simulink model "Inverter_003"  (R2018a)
settings: Solver=FixedStepDiscrete  StartTime=0.0  StopTime=inf  RelTol=1e-3  EnableMultiTasking=on
PreLoadFcn:
  | Sample_Time
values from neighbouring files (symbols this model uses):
  C_filt = 4.7e-6 /2  /2    (= 1.175e-06)    [Sample_Time.m]
  L_filt = 10e-3  /2  *2    (= 0.01)    [Sample_Time.m]
  Tcontrol = 5e-5    (= 5e-05)    [Sample_Time.m]
  Tmeasure = 5e-5     *2    (= 0.0001)    [Sample_Time.m]
  Tsample = 1e-6    (= 1e-06)    [Sample_Time.m]
  Tscope = Tcontrol*20    (= 0.001)    [Sample_Time.m]
  w = 2*pi*50    (= 314.159265359)    [Sample_Time.m]
undefined symbols (not defined in the file or in its folder): A, ADCIN0, ADCIN1, ADCINA0, ADCINB0, bit, C_filtEST, Compare, conversion, DCAEVT1, DCAEVT1FILT, Digital, Down, ended, Event, Filtered, GPTRIP1SEL, GPTRIP2SEL, input, Module, of, Single, start, Trip, TZ1, TZ2, Up, version, Zone
libraries: tiiqmathlib x32, simulink x16, c2802xlib x13, c2837xDlib x13, powerlib_meascontrol x4, etargetslib x4, c28xdmclib x1
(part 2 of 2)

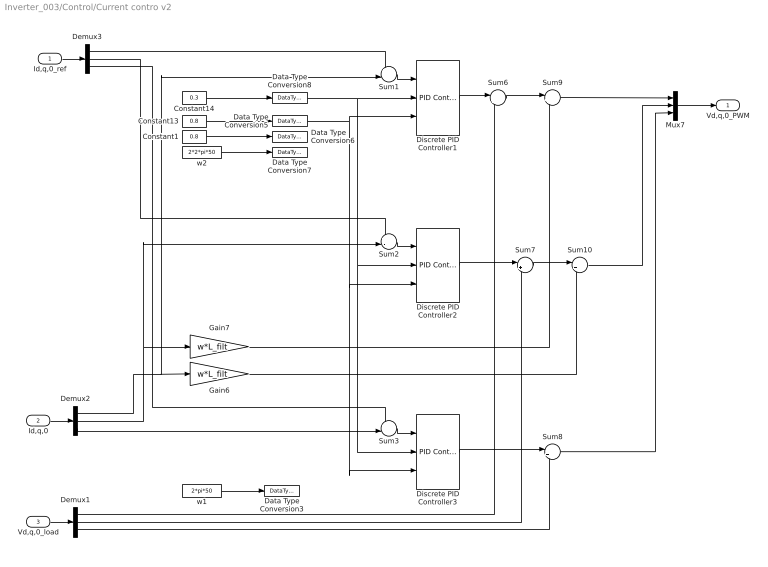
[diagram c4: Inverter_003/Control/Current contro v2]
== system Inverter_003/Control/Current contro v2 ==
  Id,q,0_ref : Inport
  Id,q,0 : Inport  Port=2
  Vd,q,0_load : Inport  Port=3
  Constant1 : Constant  Value=0.8
  Constant13 : Constant  Value=0.8
  Constant14 : Constant  Value=0.3
  Data Type Conversion{3,5..8} (5 alike) : DataTypeConversion  OutDataTypeStr=single
  Demux1 : Demux  Outputs=3
  Demux2 : Demux  Outputs=3
  Demux3 : Demux  Outputs=3
  Discrete PID Controller1 : simulink/Continuous/PID Controller  Controller=PI  TimeDomain=Discrete-time  SampleTime=Tcontrol  IntegratorMethod=Backward Euler  FilterMethod=Forward Euler  Form=Parallel  UseFilter=on  ControllerParametersSource=external  P=1  I=1  D=0  N=100  InitialConditionSource=internal  InitialConditionForIntegrator=0  InitialConditionForFilter=0  ExternalReset=none  LimitOutput=on  UpperSaturationLimit=0.98  LowerSaturationLimit=0  LinearizeAsGain=off  AntiWindupMode=clamping  Kb=1  TrackingMode=off  Kt=1  PParamMin=[]  PParamMax=[]  IParamMin=[]  IParamMax=[]  DParamMin=[]  DParamMax=[]  NParamMin=[]  NParamMax=[]  KbParamMin=[]  KbParamMax=[]  KtParamMin=[]  KtParamMax=[]  POutMin=[]  POutMax=[]  IOutMin=[]  IOutMax=[]  DOutMin=[]  DOutMax=[]  NOutMin=[]  NOutMax=[]  KbOutMin=[]  KbOutMax=[]  KtOutMin=[]  KtOutMax=[]  IntegratorOutMin=[]  IntegratorOutMax=[]  FilterOutMin=[]  FilterOutMax=[]  SumOutMin=[]  SumOutMax=[]  SumI1OutMin=[]  SumI1OutMax=[]  SumI2OutMin=[]  SumI2OutMax=[]  SumI3OutMin=[]  SumI3OutMax=[]  SumDOutMin=[]  SumDOutMax=[]  SaturationOutMin=[]  SaturationOutMax=[]  IntegratorContinuousStateAttributes=''  IntegratorStateMustResolveToSignalObject=off  IntegratorRTWStateStorageClass=Auto  FilterContinuousStateAttributes=''  FilterStateMustResolveToSignalObject=off  FilterRTWStateStorageClass=Auto  DifferentiatorICPrevScaledInput=0  DifferentiatorOutMin=[]  DifferentiatorOutMax=[]  FilterDiffOutCoefMin=[]  FilterDiffOutCoefMax=[]  SumDenOutMin=[]  SumDenOutMax=[]  SumNumOutMin=[]  SumNumOutMax=[]  ReciprocalOutMin=[]  ReciprocalOutMax=[]  DivideOutMin=[]  DivideOutMax=[]  TunerSelectOption=Transfer Function Based (PID Tuner App)
  Discrete PID Controller2 : simulink/Continuous/PID Controller  Controller=PI  TimeDomain=Discrete-time  SampleTime=Tcontrol  IntegratorMethod=Backward Euler  FilterMethod=Forward Euler  Form=Parallel  UseFilter=on  ControllerParametersSource=external  P=1  I=1  D=0  N=100  InitialConditionSource=internal  InitialConditionForIntegrator=0  InitialConditionForFilter=0  ExternalReset=none  LimitOutput=on  UpperSaturationLimit=0.98  LowerSaturationLimit=0  LinearizeAsGain=off  AntiWindupMode=clamping  Kb=1  TrackingMode=off  Kt=1  PParamMin=[]  PParamMax=[]  IParamMin=[]  IParamMax=[]  DParamMin=[]  DParamMax=[]  NParamMin=[]  NParamMax=[]  KbParamMin=[]  KbParamMax=[]  KtParamMin=[]  KtParamMax=[]  POutMin=[]  POutMax=[]  IOutMin=[]  IOutMax=[]  DOutMin=[]  DOutMax=[]  NOutMin=[]  NOutMax=[]  KbOutMin=[]  KbOutMax=[]  KtOutMin=[]  KtOutMax=[]  IntegratorOutMin=[]  IntegratorOutMax=[]  FilterOutMin=[]  FilterOutMax=[]  SumOutMin=[]  SumOutMax=[]  SumI1OutMin=[]  SumI1OutMax=[]  SumI2OutMin=[]  SumI2OutMax=[]  SumI3OutMin=[]  SumI3OutMax=[]  SumDOutMin=[]  SumDOutMax=[]  SaturationOutMin=[]  SaturationOutMax=[]  IntegratorContinuousStateAttributes=''  IntegratorStateMustResolveToSignalObject=off  IntegratorRTWStateStorageClass=Auto  FilterContinuousStateAttributes=''  FilterStateMustResolveToSignalObject=off  FilterRTWStateStorageClass=Auto  DifferentiatorICPrevScaledInput=0  DifferentiatorOutMin=[]  DifferentiatorOutMax=[]  FilterDiffOutCoefMin=[]  FilterDiffOutCoefMax=[]  SumDenOutMin=[]  SumDenOutMax=[]  SumNumOutMin=[]  SumNumOutMax=[]  ReciprocalOutMin=[]  ReciprocalOutMax=[]  DivideOutMin=[]  DivideOutMax=[]  TunerSelectOption=Transfer Function Based (PID Tuner App)
  Discrete PID Controller3 : simulink/Continuous/PID Controller  Controller=PI  TimeDomain=Discrete-time  SampleTime=Tcontrol  IntegratorMethod=Backward Euler  FilterMethod=Forward Euler  Form=Parallel  UseFilter=on  ControllerParametersSource=external  P=1  I=1  D=0  N=100  InitialConditionSource=internal  InitialConditionForIntegrator=0  InitialConditionForFilter=0  ExternalReset=none  LimitOutput=on  UpperSaturationLimit=0.98  LowerSaturationLimit=0  LinearizeAsGain=off  AntiWindupMode=clamping  Kb=1  TrackingMode=off  Kt=1  PParamMin=[]  PParamMax=[]  IParamMin=[]  IParamMax=[]  DParamMin=[]  DParamMax=[]  NParamMin=[]  NParamMax=[]  KbParamMin=[]  KbParamMax=[]  KtParamMin=[]  KtParamMax=[]  POutMin=[]  POutMax=[]  IOutMin=[]  IOutMax=[]  DOutMin=[]  DOutMax=[]  NOutMin=[]  NOutMax=[]  KbOutMin=[]  KbOutMax=[]  KtOutMin=[]  KtOutMax=[]  IntegratorOutMin=[]  IntegratorOutMax=[]  FilterOutMin=[]  FilterOutMax=[]  SumOutMin=[]  SumOutMax=[]  SumI1OutMin=[]  SumI1OutMax=[]  SumI2OutMin=[]  SumI2OutMax=[]  SumI3OutMin=[]  SumI3OutMax=[]  SumDOutMin=[]  SumDOutMax=[]  SaturationOutMin=[]  SaturationOutMax=[]  IntegratorContinuousStateAttributes=''  IntegratorStateMustResolveToSignalObject=off  IntegratorRTWStateStorageClass=Auto  FilterContinuousStateAttributes=''  FilterStateMustResolveToSignalObject=off  FilterRTWStateStorageClass=Auto  DifferentiatorICPrevScaledInput=0  DifferentiatorOutMin=[]  DifferentiatorOutMax=[]  FilterDiffOutCoefMin=[]  FilterDiffOutCoefMax=[]  SumDenOutMin=[]  SumDenOutMax=[]  SumNumOutMin=[]  SumNumOutMax=[]  ReciprocalOutMin=[]  ReciprocalOutMax=[]  DivideOutMin=[]  DivideOutMax=[]  TunerSelectOption=Transfer Function Based (PID Tuner App)
  Gain6 : Gain  Gain=w*L_filt
  Gain7 : Gain  Gain=w*L_filt
  Mux7 : Mux  Inputs=3
  Sum1 : Sum  Inputs=+-|
  Sum{6..8,10} (4 alike) : Sum  Inputs=|++
  Sum2 : Sum  Inputs=+-|
  Sum3 : Sum  Inputs=+-|
  Sum9 : Sum  Inputs=|+-
  w1 : Constant  Value=2*pi*50  OutDataTypeStr=fixdt(1,32,2^-15,0)  SampleTime=-1
  w2 : Constant  Value=2*2*pi*50  OutMin=[1e-4]  OutMax=[1000]  OutDataTypeStr=fixdt(1,32,2^-15,0)  SampleTime=-1
  Vd,q,0_PWM : Outport
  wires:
  Sum8/1 -> Mux7/3
  Discrete PID Controller2/1 -> Sum7/1
  Demux1/3 -> Sum8/2
  Demux3/3 -> Sum3/1
  Discrete PID Controller3/1 -> Sum8/1
  Demux1/1 -> Sum6/2
  Demux1/2 -> Sum7/2
  Sum6/1 -> Sum9/1
  Sum9/1 -> Mux7/1
  Sum7/1 -> Sum10/1
  Sum10/1 -> Mux7/2
  Gain7/1 -> Sum9/2
  Demux3/1 -> Sum1/1
  Demux3/2 -> Sum2/1
  Id,q,0/1 -> Demux2/1
  Id,q,0_ref/1 -> Demux3/1
  Vd,q,0_load/1 -> Demux1/1
  Demux2/2 -> Sum2/2, Gain7/1
  Demux2/1 -> Sum1/2, Gain6/1
  Mux7/1 -> Vd,q,0_PWM/1
  w1/1 -> Data Type Conversion3/1
  Constant14/1 -> Data Type Conversion8/1
  w2/1 -> Data Type Conversion7/1
  Constant13/1 -> Data Type Conversion5/1
  Constant1/1 -> Data Type Conversion6/1
  Gain6/1 -> Sum10/2
  Discrete PID Controller1/1 -> Sum6/1
  Data Type Conversion5/1 -> Discrete PID Controller1/3, Discrete PID Controller2/3, Discrete PID Controller3/3
  Data Type Conversion8/1 -> Discrete PID Controller1/2, Discrete PID Controller2/2, Discrete PID Controller3/2
  Sum1/1 -> Discrete PID Controller1/1
  Sum2/1 -> Discrete PID Controller2/1
  Sum3/1 -> Discrete PID Controller3/1
  Demux2/3 -> Sum3/2

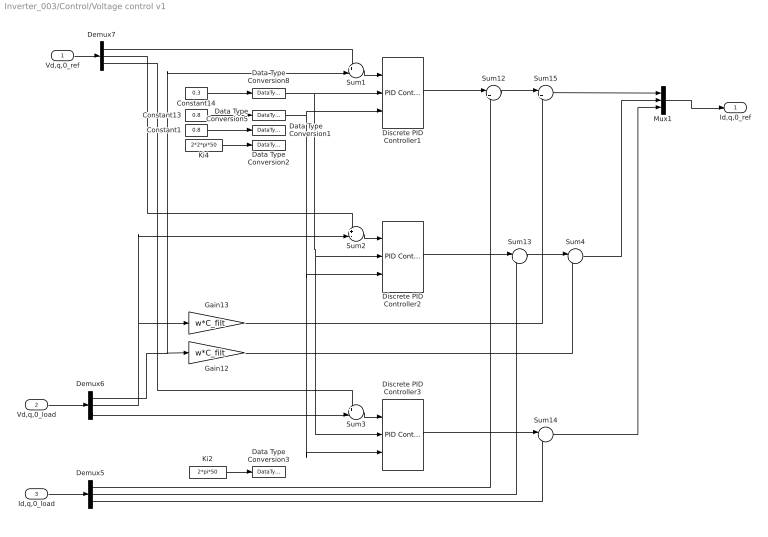
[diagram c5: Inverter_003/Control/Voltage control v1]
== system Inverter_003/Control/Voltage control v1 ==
  Vd,q,0_ref : Inport
  Vd,q,0_load : Inport  Port=2
  Id,q,0_load : Inport  Port=3
  Constant1 : Constant  Value=0.8
  Constant13 : Constant  Value=0.8
  Constant14 : Constant  Value=0.3
  Data Type Conversion{1..3,5,8} (5 alike) : DataTypeConversion  OutDataTypeStr=single
  Demux5 : Demux  Outputs=3
  Demux6 : Demux  Outputs=3
  Demux7 : Demux  Outputs=3
  Discrete PID Controller1 : simulink/Continuous/PID Controller  Controller=PI  TimeDomain=Discrete-time  SampleTime=Tcontrol  IntegratorMethod=Backward Euler  FilterMethod=Forward Euler  Form=Parallel  UseFilter=on  ControllerParametersSource=external  P=1  I=1  D=0  N=100  InitialConditionSource=internal  InitialConditionForIntegrator=0  InitialConditionForFilter=0  ExternalReset=none  LimitOutput=on  UpperSaturationLimit=0.98  LowerSaturationLimit=0  LinearizeAsGain=off  AntiWindupMode=clamping  Kb=1  TrackingMode=off  Kt=1  PParamMin=[]  PParamMax=[]  IParamMin=[]  IParamMax=[]  DParamMin=[]  DParamMax=[]  NParamMin=[]  NParamMax=[]  KbParamMin=[]  KbParamMax=[]  KtParamMin=[]  KtParamMax=[]  POutMin=[]  POutMax=[]  IOutMin=[]  IOutMax=[]  DOutMin=[]  DOutMax=[]  NOutMin=[]  NOutMax=[]  KbOutMin=[]  KbOutMax=[]  KtOutMin=[]  KtOutMax=[]  IntegratorOutMin=[]  IntegratorOutMax=[]  FilterOutMin=[]  FilterOutMax=[]  SumOutMin=[]  SumOutMax=[]  SumI1OutMin=[]  SumI1OutMax=[]  SumI2OutMin=[]  SumI2OutMax=[]  SumI3OutMin=[]  SumI3OutMax=[]  SumDOutMin=[]  SumDOutMax=[]  SaturationOutMin=[]  SaturationOutMax=[]  IntegratorContinuousStateAttributes=''  IntegratorStateMustResolveToSignalObject=off  IntegratorRTWStateStorageClass=Auto  FilterContinuousStateAttributes=''  FilterStateMustResolveToSignalObject=off  FilterRTWStateStorageClass=Auto  DifferentiatorICPrevScaledInput=0  DifferentiatorOutMin=[]  DifferentiatorOutMax=[]  FilterDiffOutCoefMin=[]  FilterDiffOutCoefMax=[]  SumDenOutMin=[]  SumDenOutMax=[]  SumNumOutMin=[]  SumNumOutMax=[]  ReciprocalOutMin=[]  ReciprocalOutMax=[]  DivideOutMin=[]  DivideOutMax=[]  TunerSelectOption=Transfer Function Based (PID Tuner App)
  Discrete PID Controller2 : simulink/Continuous/PID Controller  Controller=PI  TimeDomain=Discrete-time  SampleTime=Tcontrol  IntegratorMethod=Backward Euler  FilterMethod=Forward Euler  Form=Parallel  UseFilter=on  ControllerParametersSource=external  P=1  I=1  D=0  N=100  InitialConditionSource=internal  InitialConditionForIntegrator=0  InitialConditionForFilter=0  ExternalReset=none  LimitOutput=on  UpperSaturationLimit=0.98  LowerSaturationLimit=0  LinearizeAsGain=off  AntiWindupMode=clamping  Kb=1  TrackingMode=off  Kt=1  PParamMin=[]  PParamMax=[]  IParamMin=[]  IParamMax=[]  DParamMin=[]  DParamMax=[]  NParamMin=[]  NParamMax=[]  KbParamMin=[]  KbParamMax=[]  KtParamMin=[]  KtParamMax=[]  POutMin=[]  POutMax=[]  IOutMin=[]  IOutMax=[]  DOutMin=[]  DOutMax=[]  NOutMin=[]  NOutMax=[]  KbOutMin=[]  KbOutMax=[]  KtOutMin=[]  KtOutMax=[]  IntegratorOutMin=[]  IntegratorOutMax=[]  FilterOutMin=[]  FilterOutMax=[]  SumOutMin=[]  SumOutMax=[]  SumI1OutMin=[]  SumI1OutMax=[]  SumI2OutMin=[]  SumI2OutMax=[]  SumI3OutMin=[]  SumI3OutMax=[]  SumDOutMin=[]  SumDOutMax=[]  SaturationOutMin=[]  SaturationOutMax=[]  IntegratorContinuousStateAttributes=''  IntegratorStateMustResolveToSignalObject=off  IntegratorRTWStateStorageClass=Auto  FilterContinuousStateAttributes=''  FilterStateMustResolveToSignalObject=off  FilterRTWStateStorageClass=Auto  DifferentiatorICPrevScaledInput=0  DifferentiatorOutMin=[]  DifferentiatorOutMax=[]  FilterDiffOutCoefMin=[]  FilterDiffOutCoefMax=[]  SumDenOutMin=[]  SumDenOutMax=[]  SumNumOutMin=[]  SumNumOutMax=[]  ReciprocalOutMin=[]  ReciprocalOutMax=[]  DivideOutMin=[]  DivideOutMax=[]  TunerSelectOption=Transfer Function Based (PID Tuner App)
  Discrete PID Controller3 : simulink/Continuous/PID Controller  Controller=PI  TimeDomain=Discrete-time  SampleTime=Tcontrol  IntegratorMethod=Backward Euler  FilterMethod=Forward Euler  Form=Parallel  UseFilter=on  ControllerParametersSource=external  P=1  I=1  D=0  N=100  InitialConditionSource=internal  InitialConditionForIntegrator=0  InitialConditionForFilter=0  ExternalReset=none  LimitOutput=on  UpperSaturationLimit=0.98  LowerSaturationLimit=0  LinearizeAsGain=off  AntiWindupMode=clamping  Kb=1  TrackingMode=off  Kt=1  PParamMin=[]  PParamMax=[]  IParamMin=[]  IParamMax=[]  DParamMin=[]  DParamMax=[]  NParamMin=[]  NParamMax=[]  KbParamMin=[]  KbParamMax=[]  KtParamMin=[]  KtParamMax=[]  POutMin=[]  POutMax=[]  IOutMin=[]  IOutMax=[]  DOutMin=[]  DOutMax=[]  NOutMin=[]  NOutMax=[]  KbOutMin=[]  KbOutMax=[]  KtOutMin=[]  KtOutMax=[]  IntegratorOutMin=[]  IntegratorOutMax=[]  FilterOutMin=[]  FilterOutMax=[]  SumOutMin=[]  SumOutMax=[]  SumI1OutMin=[]  SumI1OutMax=[]  SumI2OutMin=[]  SumI2OutMax=[]  SumI3OutMin=[]  SumI3OutMax=[]  SumDOutMin=[]  SumDOutMax=[]  SaturationOutMin=[]  SaturationOutMax=[]  IntegratorContinuousStateAttributes=''  IntegratorStateMustResolveToSignalObject=off  IntegratorRTWStateStorageClass=Auto  FilterContinuousStateAttributes=''  FilterStateMustResolveToSignalObject=off  FilterRTWStateStorageClass=Auto  DifferentiatorICPrevScaledInput=0  DifferentiatorOutMin=[]  DifferentiatorOutMax=[]  FilterDiffOutCoefMin=[]  FilterDiffOutCoefMax=[]  SumDenOutMin=[]  SumDenOutMax=[]  SumNumOutMin=[]  SumNumOutMax=[]  ReciprocalOutMin=[]  ReciprocalOutMax=[]  DivideOutMin=[]  DivideOutMax=[]  TunerSelectOption=Transfer Function Based (PID Tuner App)
  Gain12 : Gain  Gain=w*C_filt
  Gain13 : Gain  Gain=w*C_filt
  Ki2 : Constant  Value=2*pi*50  OutDataTypeStr=fixdt(1,32,2^-10,0)  SampleTime=-1
  Ki4 : Constant  Value=2*2*pi*50  OutDataTypeStr=fixdt(1,32,2^-10,0)  SampleTime=-1
  Mux1 : Mux  Inputs=3
  Sum1 : Sum  Inputs=+-|
  Sum{4,12..14} (4 alike) : Sum  Inputs=|++
  Sum15 : Sum  Inputs=|+-
  Sum2 : Sum  Inputs=+-|
  Sum3 : Sum  Inputs=+-|
  Id,q,0_ref : Outport
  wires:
  Vd,q,0_load/1 -> Demux6/1
  Vd,q,0_ref/1 -> Demux7/1
  Id,q,0_load/1 -> Demux5/1
  Demux6/1 -> Sum1/2, Gain12/1
  Demux6/2 -> Sum2/2, Gain13/1
  Demux7/2 -> Sum2/1
  Demux7/1 -> Sum1/1
  Gain13/1 -> Sum15/2
  Gain12/1 -> Sum4/2
  Sum4/1 -> Mux1/2
  Sum13/1 -> Sum4/1
  Sum15/1 -> Mux1/1
  Sum12/1 -> Sum15/1
  Demux5/2 -> Sum13/2
  Demux5/1 -> Sum12/2
  Discrete PID Controller1/1 -> Sum12/1
  Discrete PID Controller3/1 -> Sum14/1
  Demux6/3 -> Sum3/2
  Demux7/3 -> Sum3/1
  Demux5/3 -> Sum14/2
  Discrete PID Controller2/1 -> Sum13/1
  Sum14/1 -> Mux1/3
  Mux1/1 -> Id,q,0_ref/1
  Constant13/1 -> Data Type Conversion5/1
  Data Type Conversion8/1 -> Discrete PID Controller1/2, Discrete PID Controller3/2, Discrete PID Controller2/2
  Data Type Conversion5/1 -> Discrete PID Controller1/3, Discrete PID Controller3/3, Discrete PID Controller2/3
  Constant1/1 -> Data Type Conversion1/1
  Ki4/1 -> Data Type Conversion2/1
  Ki2/1 -> Data Type Conversion3/1
  Sum1/1 -> Discrete PID Controller1/1
  Sum2/1 -> Discrete PID Controller2/1
  Sum3/1 -> Discrete PID Controller3/1
  Constant14/1 -> Data Type Conversion8/1

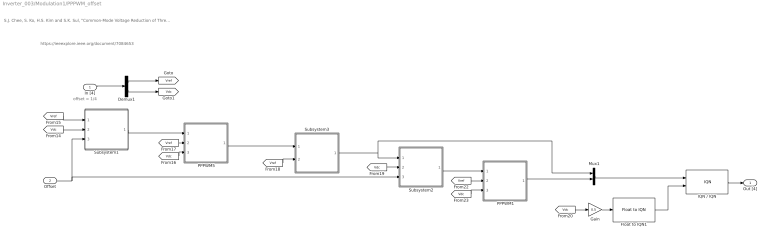
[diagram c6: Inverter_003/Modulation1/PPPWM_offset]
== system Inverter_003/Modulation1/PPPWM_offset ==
  note: offset = 1/4
  note: https://ieeexplore.ieee.org/document/7084653
  note: S.J. Chee, S. Ko, H.S. Kim and S.K. Sul, "Common-Mode Voltage Reduction of Three-Level Four-Leg PWM Converter", IEEE Transactions on Industry Applications, vol. 51, no. 5, Sept.-Oct. 2015, pp. 4006-4016
  In [4] : Inport
  Offset : Inport  Port=2
  Demux1 : Demux  Outputs=[3 1]
  Float to IQN1 : tiiqmathlib/Float to IQN  Q_value=10
  Gain : Gain  Gain=0.5  OutDataTypeStr=single
  IQN / IQN : tiiqmathlib/IQN // IQN
  Mux1 : Mux  Inputs=2
  PPPWM1 : Subsystem  TreatAsAtomicUnit=on
  PPPWM5 : Subsystem  TreatAsAtomicUnit=on
  Subsystem1 : Subsystem  TreatAsAtomicUnit=on
  Subsystem2 : Subsystem  TreatAsAtomicUnit=on
  Subsystem3 : Subsystem  TreatAsAtomicUnit=on
  Out [4] : Outport
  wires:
  Subsystem3/1(Vref *) -> Subsystem2/1(Voltage), Mux1/1
  PPPWM1/1(Vfn) -> Mux1/2
  Mux1/1 -> IQN / IQN/1
  IQN / IQN/1 -> Out [4]/1
  [Vdc] -> Gain/1
  [Vdc] -> PPPWM1/3(Vdc)
  [Vref] -> PPPWM1/2(Vref)
  Subsystem2/1(Voltage+Offset) -> PPPWM1/1(Voffset)
  PPPWM5/1(Vfn) -> Subsystem3/1(Vfn)
  [Vdc] -> Subsystem2/2(Vdc)
  [Vref] -> Subsystem3/2(Vref)
  [Vdc] -> PPPWM5/3(Vdc)
  [Vref] -> PPPWM5/2(Vref)
  [Vdc] -> Subsystem1/2(Vdc)
  [Vref] -> Subsystem1/1(Voltage)
  Demux1/2 -> [Vdc]
  Demux1/1 -> [Vref]
  Offset/1 -> Subsystem2/3(Offset), Subsystem1/3(Offset)
  In [4]/1 -> Demux1/1
  Gain/1 -> Float to IQN1/1
  Float to IQN1/1 -> IQN / IQN/2
  Subsystem1/1(Voltage+Offset) -> PPPWM5/1(Voffset)

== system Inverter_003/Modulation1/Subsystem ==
  note: Carrier
  Vref : Inport
  Add1 : Sum  Inputs=|++
  Constant : Constant  Value=-0.5  OutDataTypeStr=fixdt(1,32,2^-10,0)
  IQN1 x IQN2 : tiiqmathlib/IQN1 x IQN2  Q=10
  MinMax : MinMax  ZeroCross=off
  MinMax1 : MinMax  Function=max  ZeroCross=off
  Mux1 : Mux  Inputs=2
  Sum : Sum  Inputs=|++
  Out[4] : Outport
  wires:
  IQN1 x IQN2/1 -> Add1/2, Mux1/2  "PhaseN"
  Add1/1 -> Mux1/1
  Mux1/1 -> Out[4]/1
  Constant/1 -> IQN1 x IQN2/2
  Sum/1 -> IQN1 x IQN2/1
  Vref/1 -> MinMax/1, MinMax1/1, Add1/1
  MinMax1/1 -> Sum/2
  MinMax/1 -> Sum/1

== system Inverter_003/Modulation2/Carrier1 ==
  In1 : Inport
  Gain : Gain  Gain=-0.5
  Gain1 : Gain  Gain=-0.5
  MATLAB Function : MATLAB Function  Commented=on  TreatAsAtomicUnit=on
  MinMax : MinMax  ZeroCross=off
  MinMax1 : MinMax  Function=max  ZeroCross=off
  Sum : Sum  Inputs=|++
  Out1 : Outport
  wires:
  Sum/1 -> Out1/1
  In1/1 -> MinMax1/1, MinMax/1
  Gain1/1 -> Sum/2
  Gain/1 -> Sum/1
  MinMax1/1 -> Gain1/1, MATLAB Function/2(In2)
  MinMax/1 -> Gain/1, MATLAB Function/1(In1)

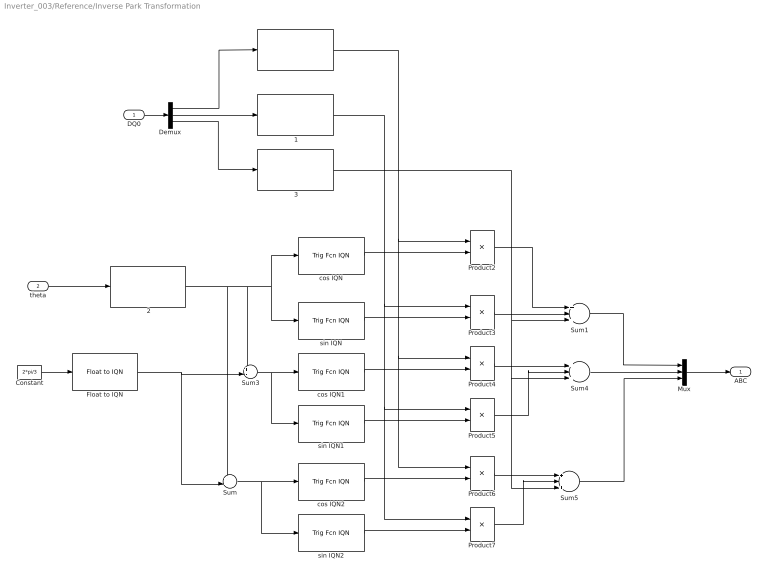
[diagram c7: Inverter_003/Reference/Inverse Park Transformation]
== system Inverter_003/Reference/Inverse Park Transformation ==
  DQ0 : Inport
  theta : Inport  Port=2
   {,1..3} (4 alike) : etargetslib/ 
  Constant : Constant  Value=2*pi/3  OutDataTypeStr=single  SampleTime=0.1
  Demux : Demux  Outputs=3
  Float to IQN : tiiqmathlib/Float to IQN  Q_value=10
  Mux : Mux  Inputs=3
  Product{2..7} (6 alike) : Product
  Sum : Sum  Inputs=++|
  Sum1 : Sum  Inputs=+-+
  Sum3 : Sum  Inputs=+-|
  Sum4 : Sum  Inputs=+-+
  Sum5 : Sum  Inputs=+-+
  cos IQN : tiiqmathlib/Trig Fcn IQN  functionOption=_IQcos
  cos IQN1 : tiiqmathlib/Trig Fcn IQN  functionOption=_IQcos
  cos IQN2 : tiiqmathlib/Trig Fcn IQN  functionOption=_IQcos
  sin IQN : tiiqmathlib/Trig Fcn IQN  functionOption=_IQsin
  sin IQN1 : tiiqmathlib/Trig Fcn IQN  functionOption=_IQsin
  sin IQN2 : tiiqmathlib/Trig Fcn IQN  functionOption=_IQsin
  ABC : Outport
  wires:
  " 2"/1 -> sin IQN/1, cos IQN/1, Sum3/1, Sum/1
  " 1"/1 -> Product7/1, Product5/1, Product3/1
  Product2/1 -> Sum1/1
  Product3/1 -> Sum1/2
  sin IQN/1 -> Product3/2
  cos IQN/1 -> Product2/2
  Demux/2 -> " 1"/1
  Demux/1 -> " "/1
  theta/1 -> " 2"/1
  Demux/3 -> " 3"/1
  Constant/1 -> Float to IQN/1
  Float to IQN/1 -> Sum/2, Sum3/2
  " 3"/1 -> Sum5/3, Sum4/3, Sum1/3
  Sum3/1 -> sin IQN1/1, cos IQN1/1
  cos IQN1/1 -> Product4/2
  sin IQN1/1 -> Product5/2
  Product4/1 -> Sum4/1
  Product5/1 -> Sum4/2
  Sum4/1 -> Mux/2
  Sum/1 -> sin IQN2/1, cos IQN2/1
  " "/1 -> Product2/1, Product4/1, Product6/1
  cos IQN2/1 -> Product6/2
  sin IQN2/1 -> Product7/2
  Product6/1 -> Sum5/1
  Product7/1 -> Sum5/2
  Sum5/1 -> Mux/3
  DQ0/1 -> Demux/1
  Sum1/1 -> Mux/1
  Mux/1 -> ABC/1

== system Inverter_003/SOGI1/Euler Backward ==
  In : Inport
  Gain1 : Gain
  Gain4 : Gain  Gain=SampleTime
  Saturation : Saturate  UpperLimit=UpperLimit  LowerLimit=LowerLimit
  Sum2 : Sum  Inputs=-+
  Sum3 : Sum  Inputs=|++
  Sum5 : Sum  Inputs=|++
  Unit Delay1 : UnitDelay  SampleTime=-1
  Unit Delay2 : UnitDelay  SampleTime=-1
  Out : Outport
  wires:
  Sum5/1 -> Saturation/1, Sum2/1, Unit Delay2/1
  Sum2/1 -> Unit Delay1/1
  Gain4/1 -> Sum3/1
  Unit Delay1/1 -> Gain1/1
  In/1 -> Gain4/1
  Saturation/1 -> Out/1, Sum2/2
  Gain1/1 -> Sum3/2
  Sum3/1 -> Sum5/1
  Unit Delay2/1 -> Sum5/2

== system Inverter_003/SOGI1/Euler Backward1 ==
  In : Inport
  Gain1 : Gain
  Gain4 : Gain  Gain=SampleTime
  Saturation : Saturate  UpperLimit=UpperLimit  LowerLimit=LowerLimit
  Sum2 : Sum  Inputs=-+
  Sum3 : Sum  Inputs=|++
  Sum5 : Sum  Inputs=|++
  Unit Delay1 : UnitDelay  SampleTime=-1
  Unit Delay2 : UnitDelay  SampleTime=-1
  Out : Outport
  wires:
  Unit Delay2/1 -> Sum5/2
  Sum3/1 -> Sum5/1
  Gain1/1 -> Sum3/2
  Saturation/1 -> Sum2/2, Out/1
  In/1 -> Gain4/1
  Unit Delay1/1 -> Gain1/1
  Gain4/1 -> Sum3/1
  Sum2/1 -> Unit Delay1/1
  Sum5/1 -> Unit Delay2/1, Sum2/1, Saturation/1

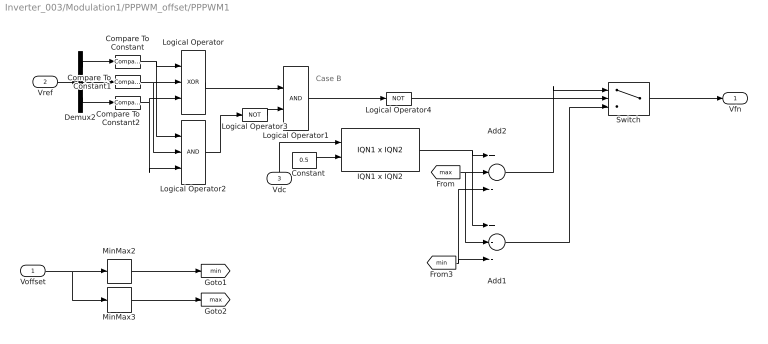
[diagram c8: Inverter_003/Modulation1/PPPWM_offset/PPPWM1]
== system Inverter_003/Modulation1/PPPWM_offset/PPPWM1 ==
  note: Case B
  Voffset : Inport
  Vref : Inport  Port=2
  Vdc : Inport  Port=3
  Add1 : Sum  Inputs=+--
  Add2 : Sum  Inputs=+--
  Compare To Constant : simulink/Logic and Bit Operations/Compare To Constant  relop=>=  const=0  OutDataTypeStr=boolean
  Compare To Constant1 : simulink/Logic and Bit Operations/Compare To Constant  relop=>=  const=0  OutDataTypeStr=boolean
  Compare To Constant2 : simulink/Logic and Bit Operations/Compare To Constant  relop=>=  const=0  OutDataTypeStr=boolean
  Constant : Constant  Value=0.5  OutDataTypeStr=fixdt(1,32,2^-10,0)
  Demux2 : Demux  Outputs=3
  IQN1 x IQN2 : tiiqmathlib/IQN1 x IQN2  Q=10
  Logical Operator : Logic  Operator=XOR  Inputs=3  AllPortsSameDT=off  OutDataTypeStr=boolean
  Logical Operator1 : Logic  AllPortsSameDT=off  OutDataTypeStr=boolean
  Logical Operator2 : Logic  Inputs=3  AllPortsSameDT=off  OutDataTypeStr=boolean
  Logical Operator3 : Logic  Operator=NOT  AllPortsSameDT=off  OutDataTypeStr=boolean
  Logical Operator4 : Logic  Operator=NOT  AllPortsSameDT=off  OutDataTypeStr=boolean
  MinMax2 : MinMax
  MinMax3 : MinMax  Function=max
  Switch : Switch  Criteria=u2 > Threshold
  Vfn : Outport
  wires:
  Switch/1 -> Vfn/1
  Constant/1 -> IQN1 x IQN2/2
  Demux2/3 -> Compare To Constant2/1
  Demux2/2 -> Compare To Constant1/1
  Demux2/1 -> Compare To Constant/1
  Compare To Constant1/1 -> Logical Operator2/2, Logical Operator/2
  MinMax3/1 -> [max]
  MinMax2/1 -> [min]
  Voffset/1 -> MinMax3/1, MinMax2/1
  Vref/1 -> Demux2/1
  Vdc/1 -> IQN1 x IQN2/1
  Compare To Constant/1 -> Logical Operator2/1, Logical Operator/1
  Logical Operator2/1 -> Logical Operator3/1
  Logical Operator1/1 -> Logical Operator4/1
  Compare To Constant2/1 -> Logical Operator2/3, Logical Operator/3
  Add1/1 -> Switch/3
  [max] -> Add1/2, Add2/2
  Add2/1 -> Switch/1
  Logical Operator3/1 -> Logical Operator1/2
  [min] -> Add2/3, Add1/3
  Logical Operator/1 -> Logical Operator1/1
  Logical Operator4/1 -> Switch/2
  IQN1 x IQN2/1 -> Add2/1, Add1/1

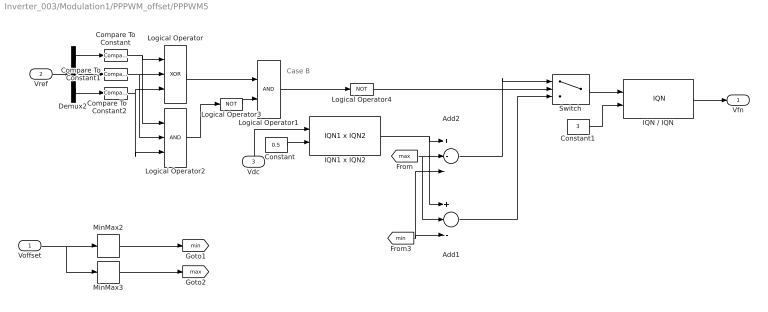
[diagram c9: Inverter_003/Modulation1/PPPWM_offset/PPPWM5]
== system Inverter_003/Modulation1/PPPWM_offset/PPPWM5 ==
  note: Case B
  Voffset : Inport
  Vref : Inport  Port=2
  Vdc : Inport  Port=3
  Add1 : Sum  Inputs=+--
  Add2 : Sum  Inputs=+--
  Compare To Constant : simulink/Logic and Bit Operations/Compare To Constant  relop=>=  const=0  OutDataTypeStr=boolean
  Compare To Constant1 : simulink/Logic and Bit Operations/Compare To Constant  relop=>=  const=0  OutDataTypeStr=boolean
  Compare To Constant2 : simulink/Logic and Bit Operations/Compare To Constant  relop=>=  const=0  OutDataTypeStr=boolean
  Constant : Constant  Value=0.5  OutDataTypeStr=fixdt(1,32,2^-10,0)
  Constant1 : Constant  Value=3  OutDataTypeStr=fixdt(1,32,2^-10,0)
  Demux2 : Demux  Outputs=3
  IQN / IQN : tiiqmathlib/IQN // IQN
  IQN1 x IQN2 : tiiqmathlib/IQN1 x IQN2  Q=10
  Logical Operator : Logic  Operator=XOR  Inputs=3  AllPortsSameDT=off  OutDataTypeStr=boolean
  Logical Operator1 : Logic  AllPortsSameDT=off  OutDataTypeStr=boolean
  Logical Operator2 : Logic  Inputs=3  AllPortsSameDT=off  OutDataTypeStr=boolean
  Logical Operator3 : Logic  Operator=NOT  AllPortsSameDT=off  OutDataTypeStr=boolean
  Logical Operator4 : Logic  Operator=NOT  AllPortsSameDT=off  OutDataTypeStr=boolean
  MinMax2 : MinMax
  MinMax3 : MinMax  Function=max
  Switch : Switch  Criteria=u2 > Threshold
  Vfn : Outport
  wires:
  IQN1 x IQN2/1 -> Add1/1, Add2/1
  Logical Operator4/1 -> Switch/2
  Logical Operator/1 -> Logical Operator1/1
  [min] -> Add1/3, Add2/3
  Logical Operator3/1 -> Logical Operator1/2
  Add2/1 -> Switch/1
  [max] -> Add2/2, Add1/2
  Add1/1 -> Switch/3
  Compare To Constant2/1 -> Logical Operator/3, Logical Operator2/3
  Logical Operator1/1 -> Logical Operator4/1
  Logical Operator2/1 -> Logical Operator3/1
  Compare To Constant/1 -> Logical Operator/1, Logical Operator2/1
  Vdc/1 -> IQN1 x IQN2/1
  Vref/1 -> Demux2/1
  Voffset/1 -> MinMax2/1, MinMax3/1
  Switch/1 -> IQN / IQN/1
  MinMax2/1 -> [min]
  MinMax3/1 -> [max]
  Compare To Constant1/1 -> Logical Operator/2, Logical Operator2/2
  Demux2/1 -> Compare To Constant/1
  Demux2/2 -> Compare To Constant1/1
  Demux2/3 -> Compare To Constant2/1
  Constant/1 -> IQN1 x IQN2/2
  IQN / IQN/1 -> Vfn/1
  Constant1/1 -> IQN / IQN/2

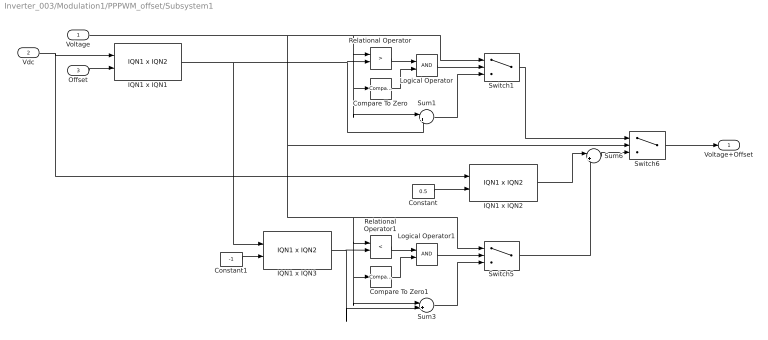
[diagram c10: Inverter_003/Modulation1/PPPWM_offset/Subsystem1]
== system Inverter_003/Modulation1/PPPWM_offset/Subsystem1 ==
  Voltage : Inport
  Vdc : Inport  Port=2
  Offset : Inport  Port=3
  Compare To Zero : simulink/Logic and Bit Operations/Compare To Zero  relop=>=  OutDataTypeStr=boolean
  Compare To Zero1 : simulink/Logic and Bit Operations/Compare To Zero  relop=<  OutDataTypeStr=boolean
  Constant : Constant  Value=0.5  OutDataTypeStr=fixdt(1,32,2^-10,0)
  Constant1 : Constant  Value=-1  OutDataTypeStr=fixdt(1,32,2^-10,0)
  IQN1 x IQN1 : tiiqmathlib/IQN1 x IQN2  Q=10
  IQN1 x IQN2 : tiiqmathlib/IQN1 x IQN2  Q=10
  IQN1 x IQN3 : tiiqmathlib/IQN1 x IQN2  Q=10
  Logical Operator : Logic  AllPortsSameDT=off  OutDataTypeStr=boolean
  Logical Operator1 : Logic  AllPortsSameDT=off  OutDataTypeStr=boolean
  Relational Operator : RelationalOperator  Operator=>  OutDataTypeStr=boolean
  Relational Operator1 : RelationalOperator  Operator=<  OutDataTypeStr=boolean
  Sum1 : Sum  Inputs=|++
  Sum3 : Sum  Inputs=|++
  Sum6 : Sum  Inputs=|++
  Switch1 : Switch  Criteria=u2 > Threshold  Threshold=0.5
  Switch5 : Switch  Criteria=u2 > Threshold  Threshold=0.5
  Switch6 : Switch
  Voltage+Offset : Outport
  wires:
  Sum6/1 -> Switch6/3
  Switch6/1 -> Voltage+Offset/1
  Voltage/1 -> Switch5/1, Compare To Zero1/1, Sum3/1, Relational Operator1/1, Switch6/2, Sum1/1, Compare To Zero/1, Relational Operator/1, Switch1/1
  Vdc/1 -> IQN1 x IQN2/1, IQN1 x IQN1/1
  Switch1/1 -> Switch6/1
  Logical Operator/1 -> Switch1/2
  Relational Operator/1 -> Logical Operator/1
  Compare To Zero/1 -> Logical Operator/2
  Sum1/1 -> Switch1/3
  IQN1 x IQN3/1 -> Sum3/2, Relational Operator1/2
  Sum3/1 -> Switch5/3
  Logical Operator1/1 -> Switch5/2
  Compare To Zero1/1 -> Logical Operator1/2
  Relational Operator1/1 -> Logical Operator1/1
  IQN1 x IQN2/1 -> Sum6/1
  IQN1 x IQN1/1 -> Relational Operator/2, Sum1/2, IQN1 x IQN3/1
  Constant/1 -> IQN1 x IQN2/2
  Offset/1 -> IQN1 x IQN1/2
  Constant1/1 -> IQN1 x IQN3/2
  Switch5/1 -> Sum6/2

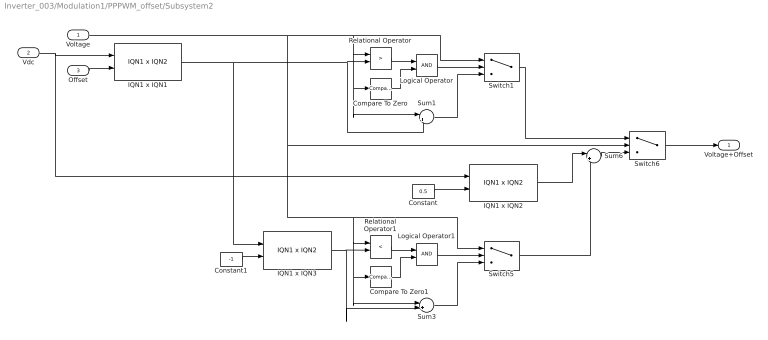
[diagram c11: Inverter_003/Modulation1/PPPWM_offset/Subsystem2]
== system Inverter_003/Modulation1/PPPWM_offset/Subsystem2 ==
  Voltage : Inport
  Vdc : Inport  Port=2
  Offset : Inport  Port=3
  Compare To Zero : simulink/Logic and Bit Operations/Compare To Zero  relop=>=  OutDataTypeStr=boolean
  Compare To Zero1 : simulink/Logic and Bit Operations/Compare To Zero  relop=<  OutDataTypeStr=boolean
  Constant : Constant  Value=0.5  OutDataTypeStr=fixdt(1,32,2^-10,0)
  Constant1 : Constant  Value=-1  OutDataTypeStr=fixdt(1,32,2^-10,0)
  IQN1 x IQN1 : tiiqmathlib/IQN1 x IQN2  Q=10
  IQN1 x IQN2 : tiiqmathlib/IQN1 x IQN2  Q=10
  IQN1 x IQN3 : tiiqmathlib/IQN1 x IQN2  Q=10
  Logical Operator : Logic  AllPortsSameDT=off  OutDataTypeStr=boolean
  Logical Operator1 : Logic  AllPortsSameDT=off  OutDataTypeStr=boolean
  Relational Operator : RelationalOperator  Operator=>  OutDataTypeStr=boolean
  Relational Operator1 : RelationalOperator  Operator=<  OutDataTypeStr=boolean
  Sum1 : Sum  Inputs=|++
  Sum3 : Sum  Inputs=|++
  Sum6 : Sum  Inputs=|++
  Switch1 : Switch  Criteria=u2 > Threshold  Threshold=0.5
  Switch5 : Switch  Criteria=u2 > Threshold  Threshold=0.5
  Switch6 : Switch
  Voltage+Offset : Outport
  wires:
  Switch5/1 -> Sum6/2
  Constant1/1 -> IQN1 x IQN3/2
  Offset/1 -> IQN1 x IQN1/2
  Constant/1 -> IQN1 x IQN2/2
  IQN1 x IQN1/1 -> IQN1 x IQN3/1, Sum1/2, Relational Operator/2
  IQN1 x IQN2/1 -> Sum6/1
  Relational Operator1/1 -> Logical Operator1/1
  Compare To Zero1/1 -> Logical Operator1/2
  Logical Operator1/1 -> Switch5/2
  Sum3/1 -> Switch5/3
  IQN1 x IQN3/1 -> Relational Operator1/2, Sum3/2
  Sum1/1 -> Switch1/3
  Compare To Zero/1 -> Logical Operator/2
  Relational Operator/1 -> Logical Operator/1
  Logical Operator/1 -> Switch1/2
  Switch1/1 -> Switch6/1
  Vdc/1 -> IQN1 x IQN1/1, IQN1 x IQN2/1
  Voltage/1 -> Switch1/1, Relational Operator/1, Compare To Zero/1, Sum1/1, Switch6/2, Relational Operator1/1, Sum3/1, Compare To Zero1/1, Switch5/1
  Switch6/1 -> Voltage+Offset/1
  Sum6/1 -> Switch6/3

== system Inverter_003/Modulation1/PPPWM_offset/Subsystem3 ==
  Vfn : Inport
  Vref : Inport  Port=2
  Sum1 : Sum  Inputs=|++
  Vref * : Outport
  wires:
  Vfn/1 -> Sum1/2
  Vref/1 -> Sum1/1
  Sum1/1 -> Vref */1

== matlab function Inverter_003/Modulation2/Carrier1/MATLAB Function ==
function y = fcn(In1, In2)

temp_min = -0.5 * In1; % min
temp_max = -0.5 * In2; % max
temp_mid = temp_min + temp_max; % min

y = temp_mid;
